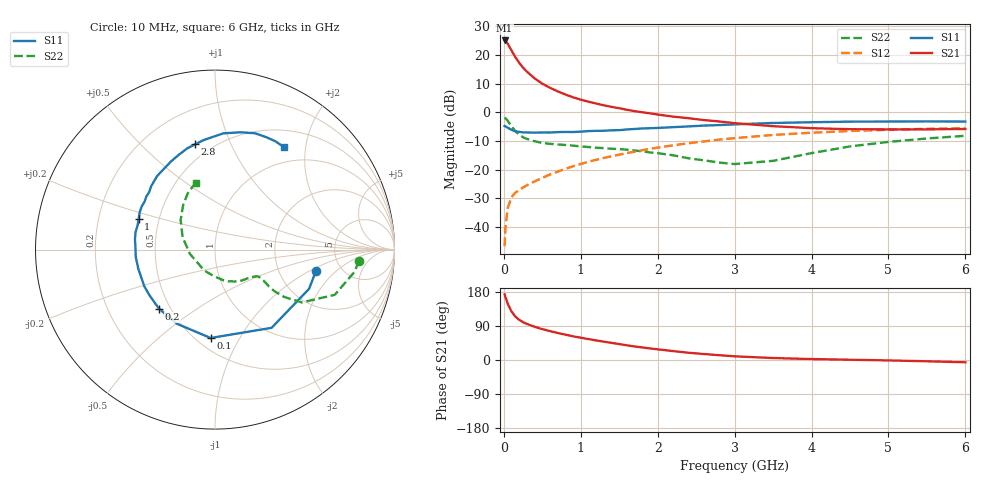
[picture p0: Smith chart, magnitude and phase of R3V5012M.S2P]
! SIEMENS Small Signal Semiconductors
! BFR181
! Si NPN RF Bipolar Junction Transistor in SOT23
! VCE = 0.5 V  IC = 12 mA
! Common Emitter S-Parameters:  May  1996
# GHz  S  MA  R  50
!  f  S11  S21  S12  S22
! GHz  MAG  ANG  MAG  ANG  MAG  ANG  MAG  ANG
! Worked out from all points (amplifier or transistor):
!   36 points, 10 MHz to 6 GHz, reference 50 ohm
!   highest |S21| = 25.1 dB at 10 MHz (marker M1)
!   |S21| within 3 dB of that: start of sweep to 89.24 MHz
!   unconditionally stable (mu >= 1): start of sweep to 15.63 MHz; 186.3 MHz to end of sweep
!   at 250 MHz: K = 1.20, MAG = 18.2 dB, |S12| = -26.2 dB
!   at 1.4 GHz: K = 1.71, MAG = 3.7 dB, |S12| = -15.4 dB
!   at 6 GHz: K = 1.23, MAG = -3.0 dB, |S12| = -5.5 dB
!   S11 on the Smith chart (normalised r, x): 10 MHz: 3.27, -1.15; 100 MHz: 0.59, -0.76; 200 MHz: 0.43, -0.36; 1 GHz: 0.38, +0.17; 2.8 GHz: 0.41, +0.74; 6 GHz: 0.74, +1.61
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0.01  0.5749 -11.8  17.89 173.1  0.0046 81.8  0.8046 -4.5
0.02  0.5681 -22.6  17.51 166.3  0.0094 79.8  0.7867 -9.1
0.05  0.5379 -54.1  15.71 148.6  0.0213 66.7  0.7134 -20.7
0.1  0.4931 -92.8  11.93 127.9  0.0329 54.9  0.5663 -31.3
0.15  0.4644 -117.0  9.132 114.5  0.0396 51.1  0.4678 -34.4
0.2  0.4537 -133.4  7.273 105.9  0.044 50.2  0.4043 -35.0
0.25  0.4451 -145.0  5.988 99.8  0.0487 50.7  0.3648 -34.4
0.3  0.4437 -152.7  5.097 95.1  0.0531 52.6  0.3425 -33.4
0.4  0.4404 -165.8  3.902 87.7  0.062 55.3  0.3116 -32.2
0.5  0.4434 -174.5  3.148 81.4  0.0716 57.7  0.2914 -31.8
0.6  0.4432 178.9  2.67 76.2  0.0819 59.3  0.2808 -32.2
0.7  0.4494 172.7  2.315 71.3  0.092 60.8  0.274 -32.9
0.8  0.4532 167.7  2.035 66.9  0.1028 60.9  0.2683 -34.1
1  0.4585 158.2  1.658 58.8  0.1251 61.7  0.2536 -37.7
1.1  0.4685 153.5  1.527 55.2  0.137 61.8  0.2473 -39.9
1.6  0.5012 135.2  1.102 38.8  0.1939 58.9  0.2223 -52.2
2.2  0.549 116.5  0.838 23.5  0.2646 52.6  0.1775 -74.5
2.8  0.597 100.6  0.69 12.7  0.3331 44.6  0.1324 -111.5
3.5  0.6494 85.9  0.571 5.2  0.4014 34.4  0.1418 -170.3
4.5  0.6854 71.0  0.506 0.7  0.4699 19.8  0.2533 139.1
5.5  0.691 60.8  0.502 -3.4  0.5135 7.3  0.3484 115.9
6  0.6881 56.3  0.51 -6.0  0.5281 1.0  0.3881 106.1
